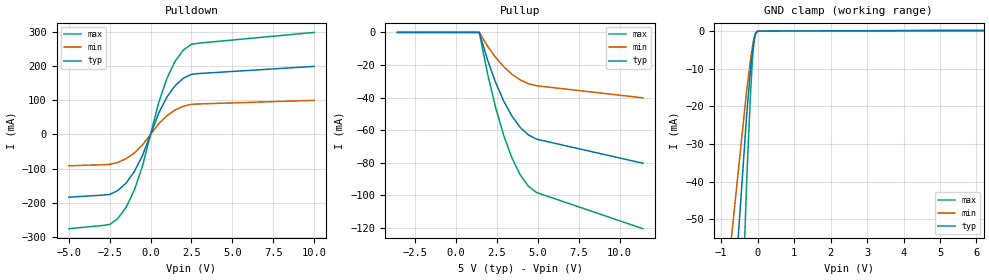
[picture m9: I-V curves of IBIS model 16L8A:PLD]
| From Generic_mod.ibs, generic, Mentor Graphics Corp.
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[Model]   16L8A:PLD
Model_type   I/O
Polarity   Non-Inverting
Vinl  =   0.800V
Vinh  =   2.000V
Vmeas =   1.500V
Cref  =  50.000pF
Rref  =   1.000kOhm
Vref  =   0.000V
|   typ   min   max
C_comp   9.000pF   4.500pF   13.500pF
[Voltage Range]   5.000V   4.500V   5.500V
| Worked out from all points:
|   slope of the pulldown table from 0 to 0.75 V, typ, clamps not added: 8.73 ohm
|   GND clamp passes 1 mA (typ) near -0.07 V on its own axis
[Pulldown]
| Voltage   I(typ)   I(min)   I(max)
-5V       -184mA     -91.98mA   -275.9mA
-2.5V     -175.8mA   -87.88mA   -263.6mA
-2V       -164.2mA   -82.09mA   -246.3mA
-1.5V     -142.6mA   -71.3mA    -213.9mA
-1V       -109.3mA   -54.66mA   -164mA
-500mV    -62.5mA    -31.25mA   -93.75mA
500mV     62.5mA     31.25mA    93.75mA
1V        109.3mA    54.66mA    164mA
1.5V      142.6mA    71.3mA     213.9mA
2V        164.2mA    82.09mA    246.3mA
3V        178mA      89.01mA    267mA
10V       198.8mA    99.42mA    298.3mA
[Pullup]
| Voltage   I(typ)   I(min)   I(max)
-3.577V   0A         0A         0A
1.423V    0A         0A         0A
1.923V    -16.67mA   -8.333mA   -25mA
2.423V    -30.7mA    -15.35mA   -46.05mA
2.923V    -42.23mA   -21.12mA   -63.35mA
3.423V    -51.38mA   -25.69mA   -77.06mA
3.923V    -58.23mA   -29.11mA   -87.34mA
4.423V    -62.89mA   -31.45mA   -94.33mA
4.923V    -65.46mA   -32.73mA   -98.19mA
11.42V    -80.28mA   -40.14mA   -120.4mA
[GND Clamp]
| Voltage   I(typ)   I(min)   I(max)
-5V       -680.2mA   -454.5mA   -1.355A
-302.9mV  -22.68mA   -16.03mA   -40.73mA
-271.5mV  -18.91mA   -13.5mA    -33.34mA
-205mV    -11.41mA   -8.406mA   -18.86mA
-165.5mV  -7.441mA   -5.668mA   -11.48mA
-134.1mV  -4.72mA    -3.743mA   -6.708mA
-110mV    -3.006mA   -2.485mA   -3.94mA
-91.21mV  -1.953mA   -1.677mA   -2.39mA
-77.65mV  -1.357mA   -1.2mA     -1.583mA
-50.74mV  -561.1uA   -523.4uA   -607.3uA
0V        0A         0A         0A
10V       128uA      128uA      128uA
[Ramp]
|   typ   min   max
dV/dt_r   1.255V/1.800ns   0.731V/3.240ns   1.675V/1.320ns
dV/dt_f   2.551V/1.500ns   1.924V/2.700ns   2.973V/1.100ns
R_load =  50.000Ohm
|------------------- End of 16L8A:PLD -----------------------------------------
